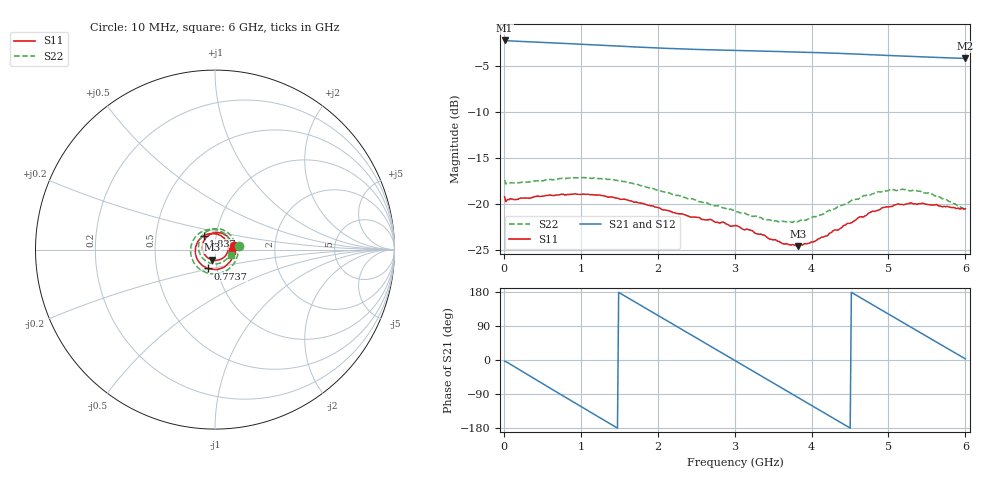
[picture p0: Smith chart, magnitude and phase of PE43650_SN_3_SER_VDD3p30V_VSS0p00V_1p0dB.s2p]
!Keysight Technologies,N5245B,MY57181451,A.13.50.07
!Date: Tuesday, May 07, 2019 07:59:46
!Correction: S11(Full 2 Port(1,2))
!S21(Full 2 Port(1,2))
!S12(Full 2 Port(1,2))
!S22(Full 2 Port(1,2))
!S2P File: Measurements: S11, S21, S12, S22:
# Hz S  dB  R 50
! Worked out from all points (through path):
!   401 points, 10 MHz to 6 GHz, reference 50 ohm
!   highest |S21| = -2.22 dB at 10 MHz (marker M1); lowest = -4.2 dB at 6 GHz (marker M2)
!   group delay of S21, straight-line fit = 331 ps
!   lowest |S11| = -24.6 dB at 3.829 GHz (marker M3), VSWR 1.12, Z = 47.9 - j5.37 ohm
!   |S11| at or under -10 dB: start of sweep to end of sweep
!   |S22| runs from -22.1 to -17.2 dB; largest |S21 - S12| = 0.0054
!   S11 on the Smith chart (normalised r, x): 10 MHz: 1.24, +0.06; 773.7 MHz: 0.90, -0.19; 1.837 GHz: 0.87, +0.13; 6 GHz: 1.21, -0.01
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1e7  -19.25 11.8  -2.22 -3.3  -2.28 -3.2  -17.41 9.5
2.1965e8  -19.39 -33.0  -2.33 -27.6  -2.38 -27.6  -17.69 -32.7
4.44275e8  -19.17 -65.6  -2.41 -55.1  -2.46 -55.1  -17.51 -65.4
7.73725e8  -18.97 -110.7  -2.53 -95.1  -2.59 -95.1  -17.24 -110.2
1.013325e9  -18.98 -141.5  -2.64 -124.1  -2.69 -124.1  -17.15 -141.0
1.432625e9  -19.34 170.5  -2.81 -174.4  -2.87 -174.4  -17.41 170.1
1.83695e9  -20.06 129.7  -2.98 137.3  -3.04 137.3  -18.15 127.0
2.01665e9  -20.46 113.1  -3.04 116.0  -3.10 116.0  -18.53 109.2
2.241275e9  -21.06 92.8  -3.12 89.3  -3.17 89.3  -19.09 87.0
2.4659e9  -21.46 71.6  -3.19 62.7  -3.24 62.7  -19.52 64.5
2.750425e9  -22.03 44.7  -3.26 29.0  -3.31 29.0  -20.22 34.5
3.005e9  -22.37 15.3  -3.31 -1.2  -3.37 -1.2  -20.76 5.2
3.45425e9  -23.85 -45.3  -3.41 -54.6  -3.45 -54.6  -21.76 -57.6
3.828625e9  -24.63 -108.1  -3.49 -99.2  -3.53 -99.2  -21.91 -117.1
4.008325e9  -24.18 -140.5  -3.53 -120.7  -3.58 -120.6  -21.50 -146.8
4.2629e9  -23.11 176.8  -3.60 -151.1  -3.65 -151.0  -20.74 173.5
4.5025e9  -22.13 141.2  -3.68 -179.7  -3.73 -179.5  -19.75 139.0
4.7421e9  -21.02 109.0  -3.77 151.8  -3.82 152.0  -19.04 108.1
5.01165e9  -20.33 78.2  -3.86 119.9  -3.91 120.0  -18.50 75.5
5.445925e9  -19.94 35.4  -4.00 68.4  -4.06 68.6  -18.85 29.0
5.745425e9  -20.34 12.5  -4.11 33.0  -4.15 33.1  -19.53 1.1
6e9  -20.55 -3.5  -4.18 2.9  -4.23 3.0  -20.73 -19.1
